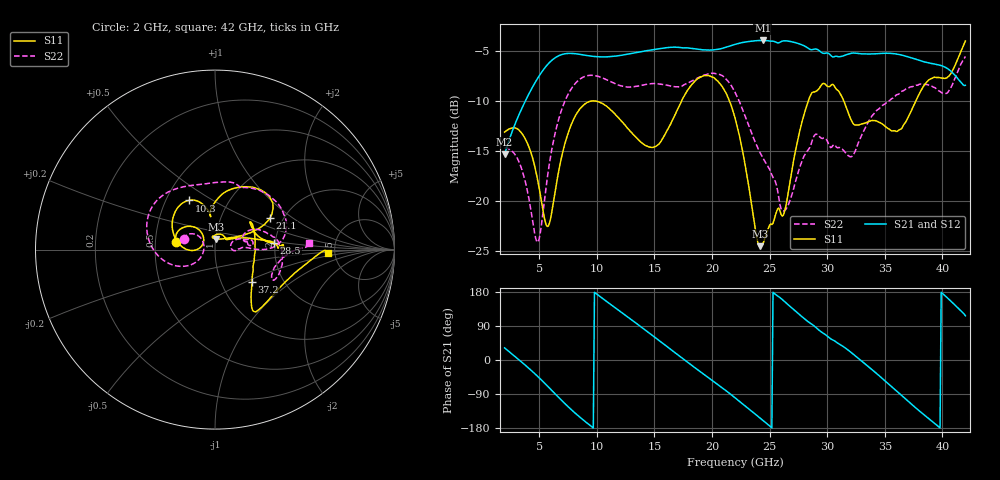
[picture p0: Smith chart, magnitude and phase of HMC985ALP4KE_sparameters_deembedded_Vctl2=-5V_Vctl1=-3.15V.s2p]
!s2p File: Measurements: S11, S21, S12, S22
# GHz S dB R 50.0
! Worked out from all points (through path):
!   401 points, 2 GHz to 42 GHz, reference 50 ohm
!   highest |S21| = -3.97 dB at 24.4 GHz (marker M1); lowest = -15.4 dB at 2 GHz (marker M2)
!   lowest |S11| = -24.5 dB at 24.2 GHz (marker M3), VSWR 1.13, Z = 50.4 + j5.97 ohm
!   |S11| at or under -10 dB: start of sweep to 17.37 GHz; 21.51 GHz to 28.37 GHz (6.856 GHz wide, 27.5 % of centre); 31.44 GHz to 37.71 GHz (6.268 GHz wide, 18.1 % of centre)
!   |S22| runs from -24.1 to -5.6 dB; largest |S21 - S12| = 0.00064
!   S11 on the Smith chart (normalised r, x): 2 GHz: 0.64, +0.06; 10.3 GHz: 0.65, +0.40; 21.1 GHz: 1.71, +0.70; 28.5 GHz: 1.97, +0.17; 37.2 GHz: 1.39, -0.55; 42 GHz: 4.38, -0.29
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2  -13.12 169.2  -15.36 32.0  -15.36 32.0  -14.70 162.1
3.4  -13.11 147.7  -10.99 -3.4  -11.00 -3.4  -16.53 143.9
4.9  -18.08 128.3  -7.68 -44.1  -7.69 -44.1  -24.10 178.5
5.8  -22.50 160.0  -6.28 -71.1  -6.29 -71.1  -16.93 -146.9
7.1  -14.86 175.7  -5.33 -111.1  -5.33 -111.1  -10.41 -170.1
8.7  -10.59 141.9  -5.38 -155.1  -5.39 -155.1  -7.70 156.2
10.3  -10.16 117.9  -5.61 167.0  -5.61 167.0  -7.62 130.8
13.1  -13.27 99.5  -5.25 104.3  -5.26 104.3  -8.60 93.6
15.4  -14.31 98.2  -4.80 51.7  -4.80 51.7  -8.31 72.4
18  -8.75 70.8  -4.72 -8.5  -4.72 -8.5  -8.17 62.1
21.1  -8.98 30.1  -4.68 -78.0  -4.68 -78.0  -7.69 16.0
22  -11.69 25.6  -4.36 -99.7  -4.37 -99.6  -9.13 4.6
24.2  -24.52 82.6  -3.97 -153.9  -3.97 -153.8  -15.23 3.8
24.4  -24.35 93.6  -3.97 -158.9  -3.97 -158.8  -15.67 4.3
26.3  -21.07 39.3  -4.00 154.2  -4.00 154.3  -20.95 12.7
28.5  -9.58 6.5  -4.85 97.8  -4.85 97.8  -14.64 17.3
28.7  -9.17 3.2  -4.89 93.8  -4.89 93.9  -13.97 16.8
32.4  -12.41 24.7  -5.23 11.8  -5.23 11.8  -15.11 26.7
35.4  -12.84 11.1  -5.25 -65.1  -5.25 -65.1  -9.98 15.1
37.2  -11.24 -41.3  -5.67 -113.4  -5.67 -113.4  -8.61 0.4
39.7  -7.66 -51.6  -6.41 -176.4  -6.41 -176.4  -9.01 -27.3
42  -4.02 -1.8  -8.45 116.7  -8.45 116.8  -5.55 3.9
